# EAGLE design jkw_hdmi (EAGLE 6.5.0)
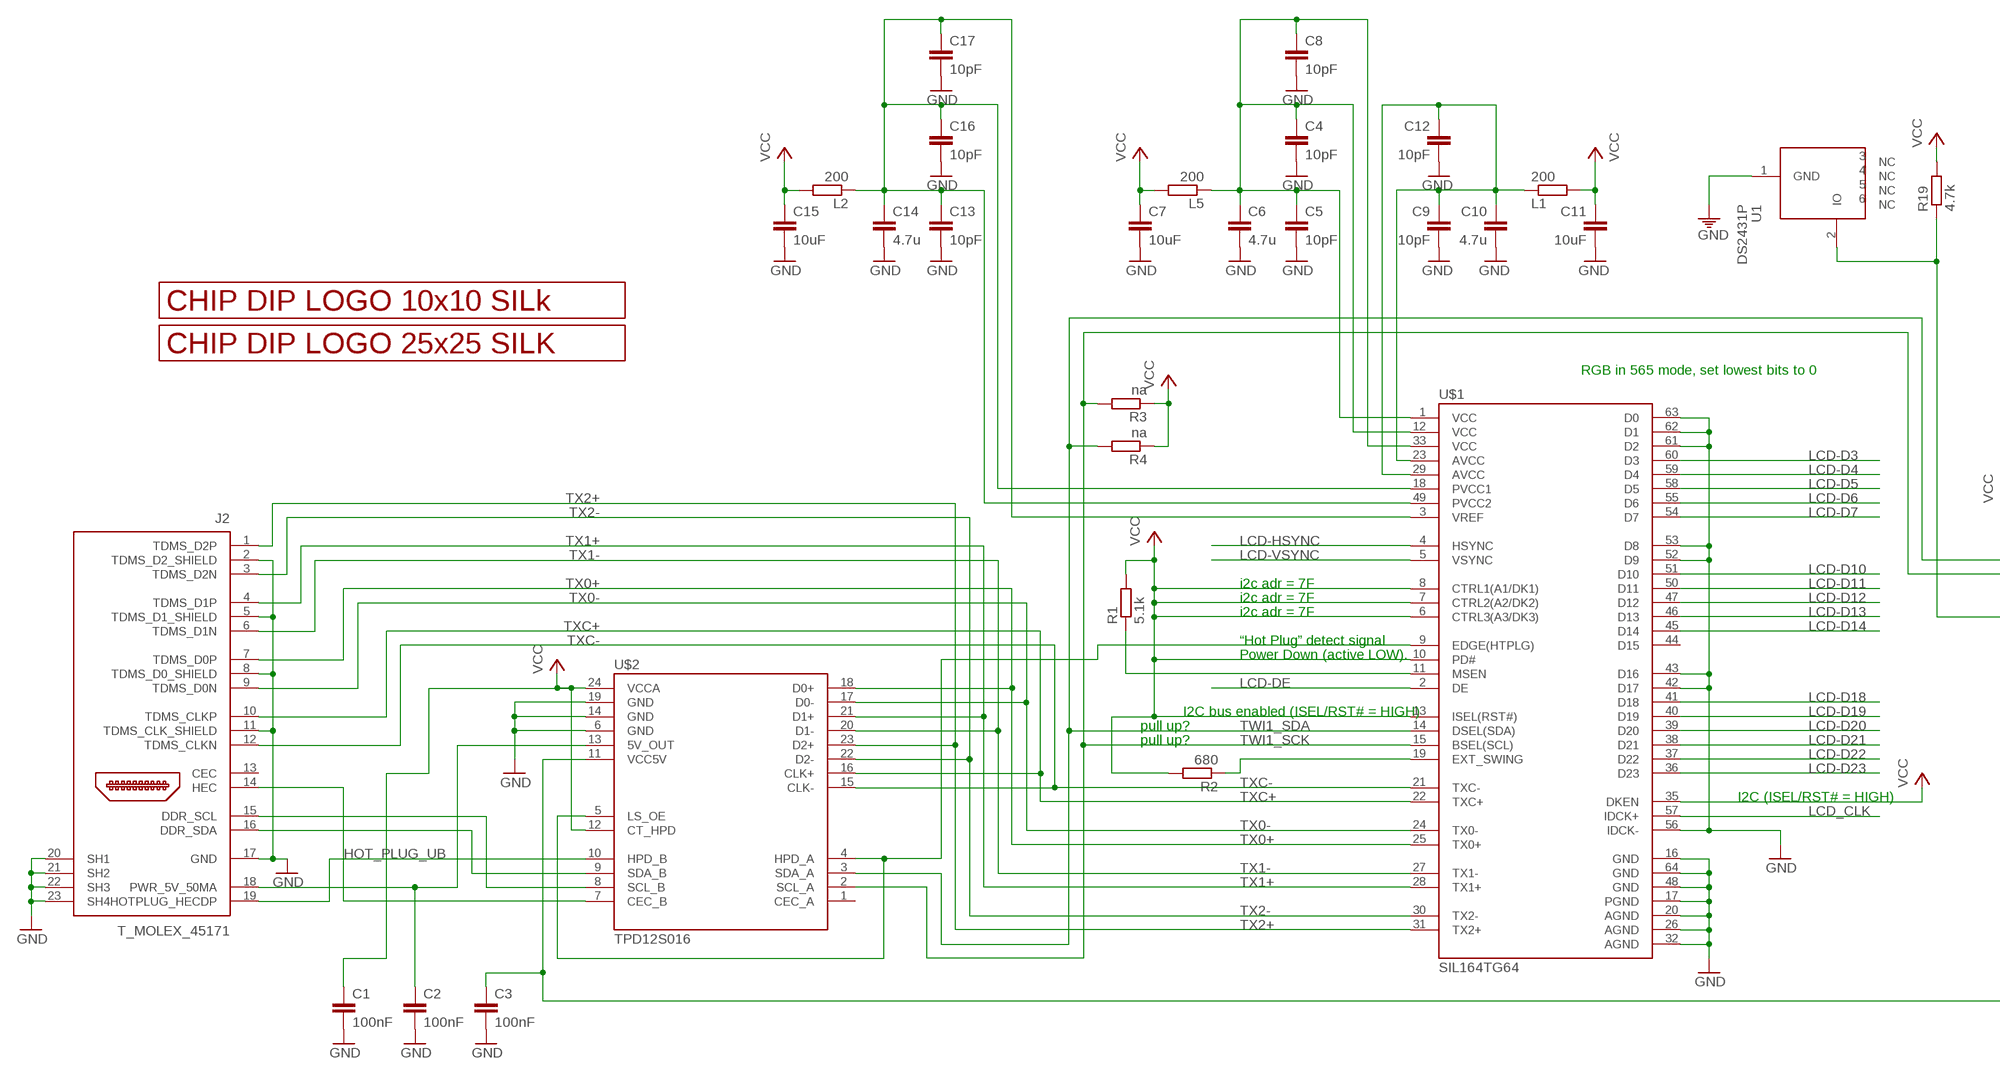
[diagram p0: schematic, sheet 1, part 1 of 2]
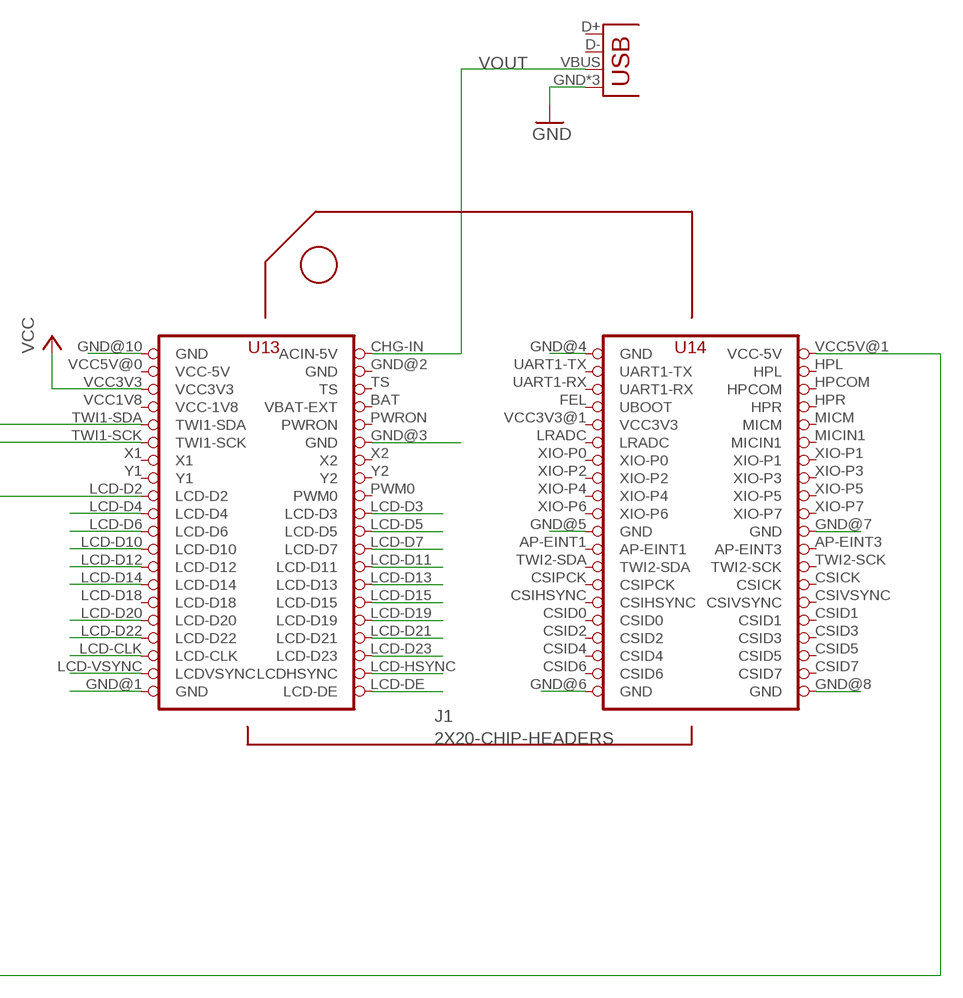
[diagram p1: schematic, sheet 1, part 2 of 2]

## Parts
C1  100nF  C-EUC0805  [C0805]
C2  100nF  C-EUC0805  [C0805]
C3  100nF  C-EUC0805  [C0805]
C4  10pF  C-EUC0805  [C0805]
C5  10pF  C-EUC0805  [C0805]
C6  4.7u  C-EUC0805  [C0805]
C7  10uF  C-EUC0805  [C0805]
C8  10pF  C-EUC0805  [C0805]
C9  10pF  C-EUC0805  [C0805]
C10  4.7u  C-EUC0805  [C0805]
C11  10uF  C-EUC0805  [C0805]
C12  10pF  C-EUC0805  [C0805]
C13  10pF  C-EUC0805  [C0805]
C14  4.7u  C-EUC0805  [C0805]
C15  10uF  C-EUC0805  [C0805]
C16  10pF  C-EUC0805  [C0805]
C17  10pF  C-EUC0805  [C0805]
J1  2X20-CHIP-HEADERS  [2X20CHIP_SM]
J2  T_MOLEX_45171  [T_MOLEX_45171]
L1  200  R-EU_R0805  [R0805]
L2  200  R-EU_R0805  [R0805]
L5  200  R-EU_R0805  [R0805]
POWER_USB  USBUSB-MICROB-SMT-DIP  [USB-MICROB-SMT-DIP]
R1  5.1k  R-EU_M0805  [M0805]
R2  680  R-EU_M0805  [M0805]
R3  na  R-EU_M0805  [M0805]
R4  na  R-EU_M0805  [M0805]
R19  4.7k  R-EU_R0805  [R0805]
U1  DS2431P  [TSOC6]
U$1  SIL164TG64  [TQFP64]
U$2  TPD12S016  [DIL24]
U$3  LOGO_10X10_SILK  [LOGO_10X10_SILK]
U$4  LOGO_25X25_SILK  [LOGO_25X25_SILK]

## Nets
ASD: R1.1 U$1.11(MSEN)
GND: C1.2 C2.2 C3.2 C4.2 C5.2 C6.2 C7.2 C8.2 C9.2 C10.2 C11.2 C12.2 C13.2 C14.2 C15.2 C16.2 C17.2 J1.GND@1(GND) J1.GND@3(GND) J1.GND@4(GND) J1.GND@5(GND) J1.GND@6(GND) J1.GND@7(GND) J1.GND@8(GND) J1.GND@10(GND) J2.2(TDMS_D2_SHIELD) J2.5(TDMS_D1_SHIELD) J2.8(TDMS_D0_SHIELD) J2.11(TDMS_CLK_SHIELD) J2.17(GND) J2.20(SH1) J2.21(SH2) J2.22(SH3) J2.23(SH4) POWER_USB.GND POWER_USB.MT1(GND) POWER_USB.MT2(GND) U1.1(GND) U$1.16(GND) U$1.17(PGND) U$1.20(AGND) U$1.26(AGND) U$1.32(AGND) U$1.42(D17) U$1.43(D16) U$1.48(GND) U$1.52(D9) U$1.53(D8) U$1.56(IDCK-) U$1.61(D2) U$1.62(D1) U$1.63(D0) U$1.64(GND) U$2.6(GND) U$2.14(GND) U$2.19(GND)
HOT_PLUG_UB: J2.19(HOTPLUG_HECDP) U$2.10(HPD_B)
HOTPLUG_DET: U$1.9(EDGE(HTPLG)) U$2.4(HPD_A) U$2.5(LS_OE)
LCD-D3: J1.LCD-D3 U$1.60(D3)
LCD-D4: J1.LCD-D4 U$1.59(D4)
LCD-D5: J1.LCD-D5 U$1.58(D5)
LCD-D6: J1.LCD-D6 U$1.55(D6)
LCD-D7: J1.LCD-D7 U$1.54(D7)
LCD-D10: J1.LCD-D10 U$1.51(D10)
LCD-D11: J1.LCD-D11 U$1.50(D11)
LCD-D12: J1.LCD-D12 U$1.47(D12)
LCD-D13: J1.LCD-D13 U$1.46(D13)
LCD-D14: J1.LCD-D14 U$1.45(D14)
LCD-D15: J1.LCD-D15
LCD-D18: U$1.41(D18)
LCD-D19: J1.LCD-D19 U$1.40(D19)
LCD-D20: J1.LCD-D20 U$1.39(D20)
LCD-D21: J1.LCD-D21 U$1.38(D21)
LCD-D22: J1.LCD-D22 U$1.37(D22)
LCD-D23: J1.LCD-D23 U$1.36(D23)
LCD-DE: J1.LCD-DE U$1.2(DE)
LCD-HSYNC: J1.LCD-HSYNC(LCDHSYNC) U$1.4(HSYNC)
LCD-VSYNC: J1.LCD-VSYNC(LCDVSYNC) U$1.5(VSYNC)
LCD_CLK: J1.LCD-CLK U$1.57(IDCK+)
N$2: R2.1 U$1.19(EXT_SWING)
N$3: C2.1 J2.18(PWR_5V_50MA) U$2.13(5V_OUT)
N$4: C4.1 C5.1 C6.1 C8.1 L5.1 U$1.1(VCC) U$1.12(VCC) U$1.33(VCC)
N$5: J1.LCD-D2 R19.1 U1.2(IO)
N$6: J2.15(DDR_SCL) U$2.8(SCL_B)
N$7: J2.16(DDR_SDA) U$2.9(SDA_B)
N$8: C9.1 C10.1 C12.1 L1.1 U$1.23(AVCC) U$1.29(AVCC)
N$9: J2.14(HEC) U$2.7(CEC_B)
N$10: C13.1 C14.1 C16.1 C17.1 L2.1 U$1.3(VREF) U$1.18(PVCC1) U$1.49(PVCC2)
TWI1_SCK: J1.TWI1-SCK R3.2 U$1.15(BSEL(SCL)) U$2.2(SCL_A)
TWI1_SDA: J1.TWI1-SDA R4.2 U$1.14(DSEL(SDA)) U$2.3(SDA_A)
TX0+: J2.7(TDMS_D0P) U$1.25(TX0+) U$2.18(D0+)
TX0-: J2.9(TDMS_D0N) U$1.24(TX0-) U$2.17(D0-)
TX1+: J2.4(TDMS_D1P) U$1.28(TX1+) U$2.21(D1+)
TX1-: J2.6(TDMS_D1N) U$1.27(TX1-) U$2.20(D1-)
TX2+: J2.1(TDMS_D2P) U$1.31(TX2+) U$2.23(D2+)
TX2-: J2.3(TDMS_D2N) U$1.30(TX2-) U$2.22(D2-)
TXC+: J2.10(TDMS_CLKP) U$1.22(TXC+) U$2.16(CLK+)
TXC-: J2.12(TDMS_CLKN) U$1.21(TXC-) U$2.15(CLK-)
VCC: C1.1 C7.1 C11.1 C15.1 J1.VCC3V3 L1.2 L2.2 L5.2 R1.2 R2.2 R3.1 R4.1 R19.2 U$1.6(CTRL3(A3/DK3)) U$1.7(CTRL2(A2/DK2)) U$1.8(CTRL1(A1/DK1)) U$1.10(PD#) U$1.13(ISEL(RST#)) U$1.35(DKEN) U$2.12(CT_HPD) U$2.24(VCCA)
VCC_5V_DCC: C3.1 J1.VCC5V@1(VCC-5V) U$2.11(VCC5V)
VOUT: J1.CHG-IN(ACIN-5V) POWER_USB.VBUS
Unconnected: J1.AP-EINT1 J1.AP-EINT3 J1.BAT(VBAT-EXT) J1.CSICK J1.CSID0 J1.CSID1 J1.CSID2 J1.CSID3 J1.CSID4 J1.CSID5 J1.CSID6 J1.CSID7 J1.CSIHSYNC J1.CSIPCK J1.CSIVSYNC J1.FEL(UBOOT) J1.HPCOM J1.HPL J1.HPR J1.LCD-D18 J1.LRADC J1.MICIN1 J1.MICM J1.PWM0 J1.PWRON J1.TS J1.TWI2-SCK J1.TWI2-SDA J1.UART1-RX J1.UART1-TX J1.X1 J1.X2 J1.XIO-P0 J1.XIO-P1 J1.XIO-P2 J1.XIO-P3 J1.XIO-P4 J1.XIO-P5 J1.XIO-P6 J1.XIO-P7 J1.Y1 J1.Y2 J2.13(CEC) POWER_USB.D+ POWER_USB.D- U1.3(NC) U1.4(NC) U1.5(NC) U1.6(NC) U$2.1(CEC_A)

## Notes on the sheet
- RGB in 565 mode, set lowest bits to 0
- i2c adr = 7F
- i2c adr = 7F
- i2c adr = 7F
- “Hot Plug” detect signal
- Power Down (active LOW).
- I2C bus enabled (ISEL/RST# = HIGH)
- pull up?
- pull up?
- I2C (ISEL/RST# = HIGH)

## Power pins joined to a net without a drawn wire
D15: U$1.44(D15)
GND: J1.GND@2(GND)
VCC3V3: J1.VCC3V3@1(VCC3V3)
VCC-1V8: J1.VCC1V8(VCC-1V8)
VCC-5V: J1.VCC5V@0(VCC-5V)

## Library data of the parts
C1-C17 = rcl:C-EU: CAPACITOR, European symbol
J1 = VGA-DIP:2X20-CHIP-HEADERS: Through hole layout with chip reference
J2 = CHIP_HDMI:T_MOLEX_45171
L1 L2 L5 R1-R4 R19 = rcl:R-EU_: RESISTOR, European symbol
POWER_USB = Spark:USB
U1 = VGA-DIP:DS2431: 1024-Bit EEPROM This chip provides a 4x256 Bit EEPROM, which can be programmed@5V. Write protection and OTP emulation are available, too. Author: Jan Kandziora <jjj@gmx.de>; DESCRIPTION: IC, 1024-Bit, 1-Wire EEPROM, TSOC6; FOOTPRINT: TSOC6; LINK: http://www.digikey.com/product-detail/en/DS2431P%2BT%26R/DS2431P%2BT%26RCT-ND/3647900; MFG: DIGIKEY; MFG_PN: DS2431P+T&RCT-ND; PART_TYPE: IC; PRICE: 0.98; VENDOR: MAXIM; VENDOR_PART_NUMBER: DS2431P+T&R
U$1 = SII164CTG64:SIL164TG64
U$2 = SII164CTG64:TPD12S016
U$3 = logo:LOGO_10X10_SILK
U$4 = logo:LOGO_25X25_SILK

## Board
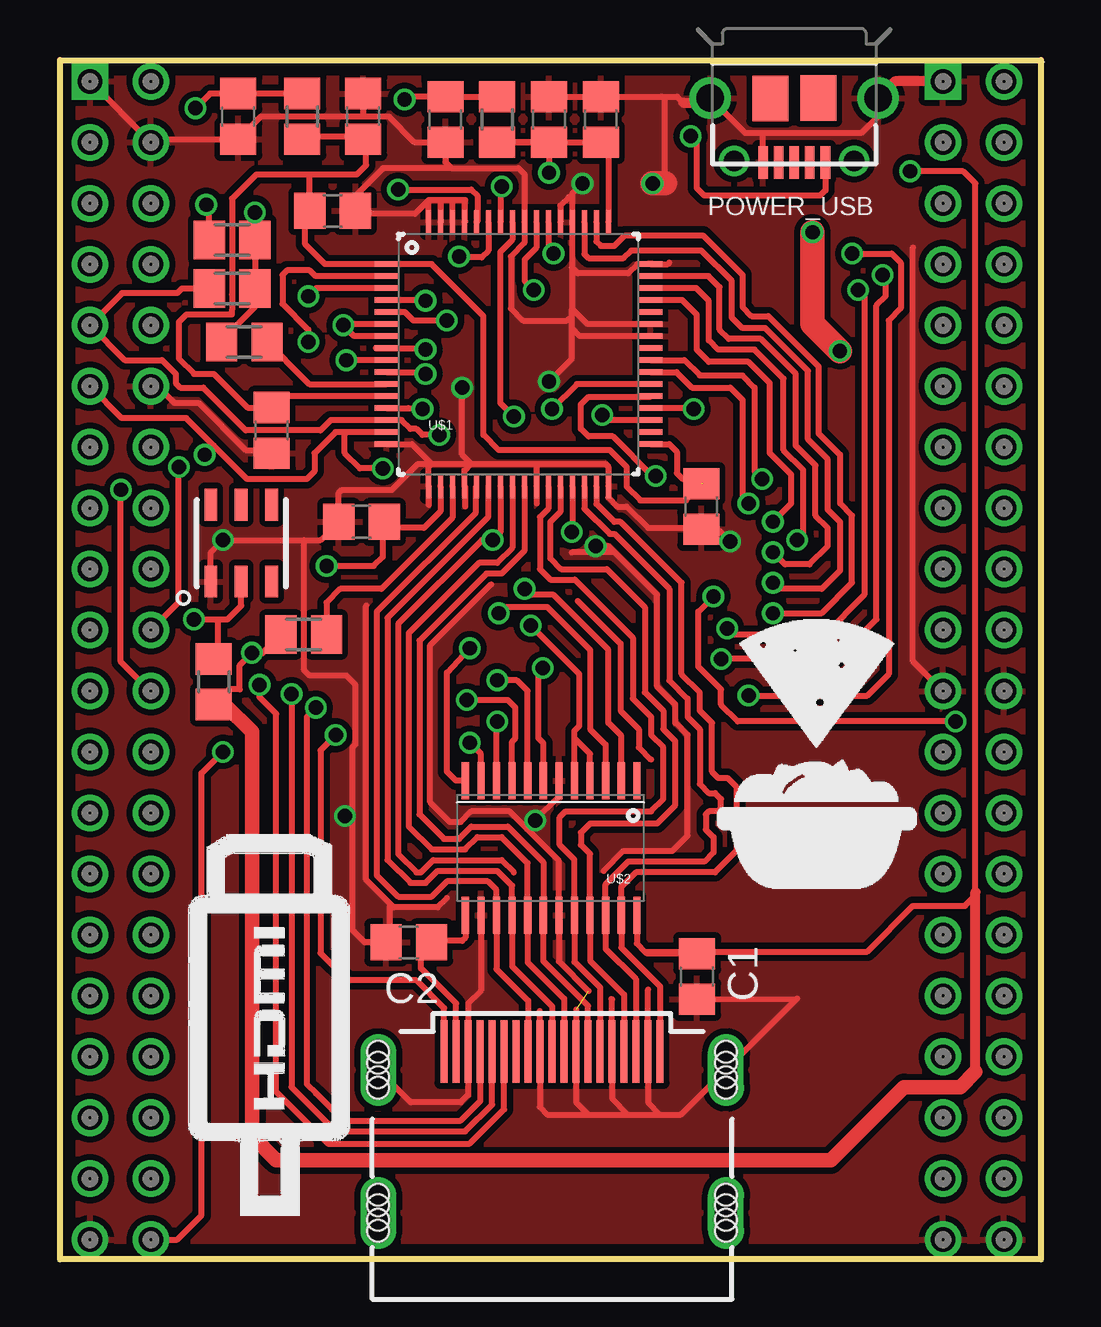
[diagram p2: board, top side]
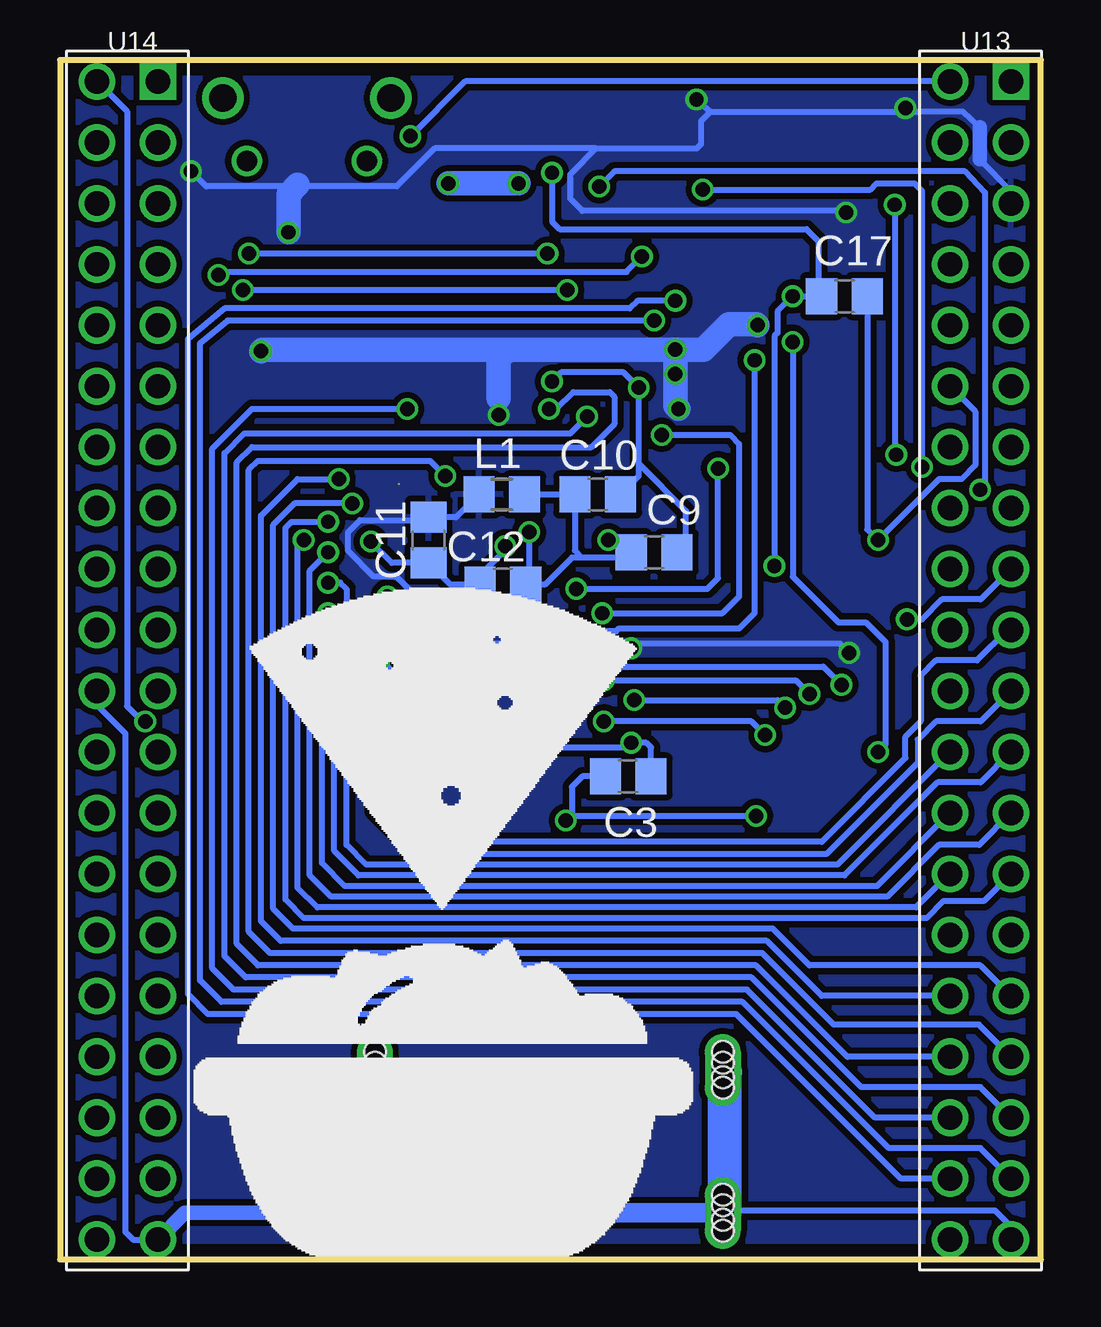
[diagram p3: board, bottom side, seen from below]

Size 40.89 x 49.97 mm. Coordinates in mm from the lower left corner, seen from the top.
Outline: 0,49.97 40.89,49.97 40.89,0 0,0 0,49.97
Copper layers (1*16): Top 0.035mm / dielectric 1.6mm / Bottom 0.035mm
Design rules "Elecrow_2-layer_PCB_eagle_rule": minimum track width 6mil, minimum drill 12mil, track to track 6mil, track to pad 6mil, pad to pad 6mil, via to via 8mil, smd to smd 0mil, copper to edge 20mil, drill to drill 10mil, minimum pad ring 6mil, minimum via ring 6mil, stop-mask expansion 0mil, vias tented up to drill 100mil, thermal gap 10mil

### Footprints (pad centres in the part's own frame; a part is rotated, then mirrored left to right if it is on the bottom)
C0805 = smd 1.3 x 1.5: 1 -0.95,0; 2 0.95,0
2X20CHIP_SM = drill 1.016: AP-EINT1 36.81,21.65; AP-EINT3 39.35,21.65; BAT 3.79,41.97; CHG-IN 3.79,49.59; CSICK 39.35,16.57; CSID0 36.81,11.49; CSID1 39.35,11.49; CSID2 36.81,8.95; CSID3 39.35,8.95; CSID4 36.81,6.41; CSID5 39.35,6.41; CSID6 36.81,3.87; CSID7 39.35,3.87; CSIHSYNC 36.81,14.03; CSIPCK 36.81,16.57; CSIVSYNC 39.35,14.03; FEL 36.81,41.97; GND@1 3.79,36.89; GND@2 1.25,1.33; GND@4 39.35,24.19; GND@5 39.35,1.33; GND@6 36.81,1.33; GND@7 36.81,24.19; GND@10 3.79,47.05; HPCOM 39.35,44.51; HPL 39.35,47.05; HPR 39.35,41.97; LCD-CLK 1.25,6.41; LCD-D2 1.25,29.27; LCD-D3 3.79,26.73; LCD-D4 1.25,26.73; LCD-D5 3.79,24.19; LCD-D6 1.25,24.19; LCD-D7 3.79,21.65; LCD-D10 1.25,21.65; LCD-D11 3.79,19.11; LCD-D12 1.25,19.11; LCD-D13 3.79,16.57; LCD-D14 1.25,16.57; LCD-D15 3.79,14.03; LCD-D18 1.25,14.03; LCD-D19 3.79,11.49; LCD-D20 1.25,11.49; LCD-D21 3.79,8.95; LCD-D22 1.25,8.95; LCD-D23 3.79,6.41; LCD-DE 3.79,1.33; LCD-HSYNC 3.79,3.87; LCD-VSYNC 1.25,3.87; LRADC 36.81,36.89; MICIN1 39.35,36.89; MICM 39.35,39.43; PWM0 3.79,29.27; PWRON 3.79,39.43; TS 3.79,44.51; TWI1-SCK 1.25,36.89; TWI1-SDA 1.25,39.43; TWI2-SCK 39.35,19.11; TWI2-SDA 36.81,19.11; UART1-RX 36.81,44.51; UART1-TX 36.81,47.05; VCC1V8 1.25,41.97; VCC3V3 1.25,44.51; VCC3V3@1 36.81,39.43; VCC5V@0 1.25,47.05; VCC5V@1 39.35,49.59; X1 1.25,34.35; X2 3.79,34.35; XIO-P0 36.81,34.35; XIO-P1 39.35,34.35; XIO-P2 36.81,31.81; XIO-P3 39.35,31.81; XIO-P4 36.81,29.27; XIO-P5 39.35,29.27; XIO-P6 36.81,26.73; XIO-P7 39.35,26.73; Y1 1.25,31.81; Y2 3.79,31.81 | drill 1.016 square: GND@3 1.25,49.59; GND@8 36.81,49.59
T_MOLEX_45171 = smd 0.3 x 2.6: 1 4.5,10.31; 2 4,10.31; 3 3.5,10.31; 4 3,10.31; 5 2.5,10.31; 6 2,10.31; 7 1.5,10.31; 8 1,10.31; 9 0.5,10.31; 10 0,10.31; 11 -0.5,10.31; 12 -1,10.31; 13 -1.5,10.31; 14 -2,10.31; 15 -2.5,10.31; 16 -3,10.31; 17 -3.5,10.31; 18 -4,10.31; 19 -4.5,10.31 | drill 0.9 pad 1.499 long: 20 -7.25,3.59; 21 7.25,3.59; 22 7.25,9.55; 23 -7.25,9.55 | hole 0.9: -7.25,10.3; -7.25,8.8; -7.25,9.85; -7.25,9.25; -7.25,4.35; -7.25,2.85; -7.25,3.9; -7.25,3.3; 7.25,10.3; 7.25,8.8; 7.25,9.85; 7.25,9.25; 7.25,4.35; 7.25,3.9; 7.25,2.85; 7.25,3.3
R0805 = smd 1.3 x 1.5: 1 -0.95,0; 2 0.95,0
USB-MICROB-SMT-DIP = smd 0.4 x 1.35: D+ 0,2.675; D- -0.65,2.675; GND 1.3,2.675; ID 0.65,2.675; VBUS -1.3,2.675 | drill 1.15 pad 1.7: MT1 -3.5,0; MT2 3.5,0 | drill 0.85 pad 1.25: MT3 -2.5,2.625; MT4 2.5,2.625 | smd 1.5 x 1.9: P$1 -1,0; P$2 1,0.01
M0805 = smd 1.3 x 1.6: 1 -0.95,0; 2 0.95,0
TSOC6 = smd 0.53 x 1.33: 1 -1.27,-1.6; 2 0,-1.6; 3 1.27,-1.6; 4 1.27,1.6; 5 0,1.6; 6 -1.27,1.6
TQFP64 = smd 1 x 0.22: 1 -5.5,3.75; 2 -5.5,3.25; 3 -5.5,2.75; 4 -5.5,2.25; 5 -5.5,1.75; 6 -5.5,1.25; 7 -5.5,0.75; 8 -5.5,0.25; 9 -5.5,-0.25; 10 -5.5,-0.75; 11 -5.5,-1.25; 12 -5.5,-1.75; 13 -5.5,-2.25; 14 -5.5,-2.75; 15 -5.5,-3.25; 16 -5.5,-3.75; 33 5.5,-3.75; 34 5.5,-3.25; 35 5.5,-2.75; 36 5.5,-2.25; 37 5.5,-1.75; 38 5.5,-1.25; 39 5.5,-0.75; 40 5.5,-0.25; 41 5.5,0.25; 42 5.5,0.75; 43 5.5,1.25; 44 5.5,1.75; 45 5.5,2.25; 46 5.5,2.75; 47 5.5,3.25; 48 5.5,3.75 | smd 0.22 x 1: 17 -3.75,-5.5; 18 -3.25,-5.5; 19 -2.75,-5.5; 20 -2.25,-5.5; 21 -1.75,-5.5; 22 -1.25,-5.5; 23 -0.75,-5.5; 24 -0.25,-5.5; 25 0.25,-5.5; 26 0.75,-5.5; 27 1.25,-5.5; 28 1.75,-5.5; 29 2.25,-5.5; 30 2.75,-5.5; 31 3.25,-5.5; 32 3.75,-5.5; 49 3.75,5.5; 50 3.25,5.5; 51 2.75,5.5; 52 2.25,5.5; 53 1.75,5.5; 54 1.25,5.5; 55 0.75,5.5; 56 0.25,5.5; 57 -0.25,5.5; 58 -0.75,5.5; 59 -1.25,5.5; 60 -1.75,5.5; 61 -2.25,5.5; 62 -2.75,5.5; 63 -3.25,5.5; 64 -3.75,5.5
DIL24 = smd 0.3 x 1.55: 1 -3.6,-2.8; 2 -2.95,-2.8; 3 -2.3,-2.8; 4 -1.65,-2.8; 5 -1,-2.8; 6 -0.35,-2.8; 7 0.3,-2.8; 8 0.95,-2.8; 9 1.6,-2.8; 10 2.25,-2.8; 11 2.9,-2.8; 12 3.55,-2.8; 13 3.55,2.8; 14 2.9,2.8; 15 2.25,2.8; 16 1.6,2.8; 17 0.95,2.8; 18 0.3,2.8; 19 -0.35,2.8; 20 -1,2.8; 21 -1.65,2.8; 22 -2.3,2.8; 23 -2.95,2.8; 24 -3.6,2.8

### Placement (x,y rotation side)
C1  26.56,11.79 270 top
C2  14.54,13.21 180 top
C3  17.21,20.13 180 bottom
C4  8.83,34.54 270 top
C5  11.37,43.69 0 top
C6  12.64,47.62 90 top
C7  7.43,47.62 270 top
C8  26.73,31.37 270 top
C9  16.13,29.46 0 bottom
C10  18.48,31.88 0 bottom
C11  25.53,29.97 270 bottom
C12  22.43,28.12 180 bottom
C13  22.54,47.5 90 top
C14  20.38,47.5 90 top
C15  16.07,47.5 270 top
C16  12.57,30.73 180 top
C17  8.19,40.13 0 bottom
J1  0,-0.51 0 top
J2  20.51,-1.65 0 top
L1  22.48,31.88 180 bottom
L2  18.22,47.5 90 top
L5  10.1,47.62 90 top
POWER_USB  30.61,48.39 180 top
R1  7.68,38.23 180 top
R2  10.16,26.04 180 top
R3  7.18,42.48 180 top
R4  7.18,40.45 180 top
R19  6.41,24.07 270 top
U1  7.56,29.84 0 top
U$1  19.11,37.72 0 top
U$2  20.45,17.15 180 top
U$3  27.37,15.43 0 top
U$4  35.37,-0.13 0 bottom

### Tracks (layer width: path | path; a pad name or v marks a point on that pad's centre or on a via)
ASD
  Top 0.254: R1.1 8.45,38.42 10.39,36.47 U$1.11
GND  (via drill 0.6)  (1 unrouted)
  Top 0.254: C14.2 C13.2 25.08,48.45 | 24.51,11.24 J2.2 24.51,6.54 25.02,6.03 | J2.11 | J2.11 20,10.35 | 21.53,10.41 21.53,8.68 J2.8 21.51,6.56 22.04,6.03 | 22.99,10.86 23.01,10.84 J2.5 23.01,6.71 23.69,6.03 | 22.04,11.18 20.8,12.41 U$2.19 20.8,16.6 19.46,17.94 | 19.88,31.5 19.88,32.21 | 19.88,32.21 U$1.26 | 17.97,28.13 15.43,25.59 15.43,19.05 16.26,18.23 16.7,18.23 17.14,18.67 18.73,18.67 19.46,17.94 | 20.83,19.91 U$2.6 20.8,19.27 v19.81,18.29 19.46,17.94 | J2.23 14.62,6.54 16.7,6.54 17.01,6.85 J2.17 17.02,10.67 17.55,11.2 U$2.14 | 25.4,41.53 25.34,41.47 U$1.48 24.07,41.47 23.69,41.09 21.59,41.09 21.34,41.34 21.36,41.37 | U$1.52 21.36,44.11 21.21,44.26 20.86,43.91 U$1.53 | U$1.61 16.89,43.25 16.89,44.13 16.32,44.13 | U$1.63 15.88,43.23 15.88,44.13 | 16.32,44.13 15.88,44.13 | 15.88,44.13 15.37,44.13 15.36,44.13 | 16.89,31.37 16.89,32.19 U$1.20 16.86,32.87 17.14,33.15 | 15.37,31.43 U$1.17 15.36,33.02 15.49,33.15 | J1.GND@1 4.07,36.38 4.76,35.69 5.78,35.69 7.75,33.72 8.7,33.72 C4.2 | 27.94,8.08 J2.22 | 19.88,32.21 19.88,33.08 19.94,33.15 | 19.94,33.15 22.73,33.15 22.86,33.02 U$1.32 22.86,31.75 23.24,31.37 23.62,31.37 24.51,30.48 26.67,30.48 C8.2 26.8,30.35 27.49,30.35 v27.94,29.91 | 17.14,33.15 19.94,33.15 | U$1.16 14.67,33.97 15.49,33.15 | U$1.64 15.36,44.13 | U$1.52 21.36,44.41 v21.78,44.83 | 21.36,41.37 U$1.52 | U$1.43 21.99,38.97 21.36,39.6 | 21.36,39.6 21.36,41.37 | U$1.42 21.67,38.47 21.34,38.8 | 21.34,38.8 21.34,39.31 | 21.34,39.31 21.34,39.57 21.36,39.6 | 17.14,33.15 16.76,33.53 v16.76,36.32 | v20.38,36.58 21.34,37.53 21.34,38.8 | 15.49,33.15 17.14,33.15 | 25.08,48.45 25.72,48.45 25.97,48.2 | 15.36,44.13 14.8,43.56 12.44,43.56 C5.2 12.32,44.32 13.46,45.47 16.32,45.47
  Top 0.254: 16.32,45.47 16.07,45.72 C15.2 14.77,46.55 13.69,47.62 12.7,47.62 | 16.32,45.47 19.11,45.47 19.37,45.21 U$1.56 19.36,42.35 18.8,41.78 18.8,39.62 19.3,39.12 21.15,39.12 21.34,39.31 | 12.7,47.62 8.38,47.62 C7.2 3.92,46.68 J1.GND@10 J1.GND@3 | C6.2 12.64,47.69 12.7,47.62 | U$1.62 16.36,44.09 16.32,44.13 | U1.1 6.29,29.46 v6.79,29.97 10.16,29.97 | 10.16,29.97 10.86,29.97 C16.2 11.62,31.94 11.75,32.07 13.84,32.07 14.92,33.15 15.49,33.15 | J2.11 20,6.35 20.32,6.03 22.04,6.03 | 22.04,6.03 23.69,6.03 | 23.69,6.03 25.02,6.03 | 25.02,6.03 25.89,6.03 J2.22 | 10.16,29.97 10.16,24.57 10.41,24.32 11.94,24.32 12.32,23.94 12.32,21.46 12.19,21.34 12.19,13.72 12.7,13.21 C2.2 13.75,13.37 13.75,14.82 | C1.2 30.72,10.86 J2.22 | J1.GND@7 35.56,24.93 35.56,42.16 | POWER_USB.MT1 34.11,47.63 33.4,46.93 29.34,46.93 | 29.34,46.93 28.57,46.93 POWER_USB.MT2 | POWER_USB.GND 29.31,46.9 29.34,46.93 | 25.21,44.83 25.21,48.32 25.08,48.45 | 16.13,15.05 15.75,14.67 13.91,14.67 13.75,14.82 | 13.75,14.82 12.76,15.81 12.76,27.24 | 22.67,16.19 23.49,17.02 25.53,17.02 26.16,17.65 26.16,21.84 25.65,22.35 25.65,23.11 24.89,23.88 24.89,27.69 23.11,29.46 | 23.11,29.46 21.34,29.46 | 23.11,29.46 22.86,29.72 v22.33,29.72
  Top 0.406: 25.97,48.2 27.11,48.2 POWER_USB.MT2 | J1.GND@8 34.8,49.08 POWER_USB.MT1
  Top 1.016: v24.7,44.83 25.21,44.83
  Bottom 0.254: J1.GND@2 1.25,1.38 1.91,2.03 13.17,2.03 J2.20 | J1.GND@6 37.85,0.82 38.16,1.14 38.16,21.91 39.35,23.09 J1.GND@4 | 13.17,7.81 J2.23 | C3.2 19.11,20.13 19.56,19.69 19.56,18.54 19.62,18.48 | v20.38,36.58 20,36.96 17.4,36.96 v16.76,36.32 16.76,33.15 | C10.2 16.76,32.64 16.76,33.15 | C9.2 14.8,29.85 14.8,31.18 16.76,33.15 | C17.2 7.24,30.42 v6.79,29.97 4.25,32.51 3.3,32.51 2.74,33.08 2.74,35.34 J1.GND@1 | 25.21,28.7 C11.2 | C11.2 27.05,29.02 v27.94,29.91 | 19.62,18.48 v19.81,18.29 | 19.62,18.48 v11.88,18.48 | 23.38,28.6 23.38,28.51 | C11.2 24.62,28.12 C12.2 23.38,28.51 | 23.38,28.51 22.33,29.56 v22.33,29.72
  Bottom 0.61: J2.21 35.69,1.94 J1.GND@6
  Bottom 0.813: J2.20 J2.21
  Bottom 1.016: v21.78,44.83 v24.7,44.83
  Bottom 1.422: J2.21 J2.22 | 13.17,2.03 13.17,7.81
  pour Top (isolate 0.254): 0.13,0 40.89,0 40.89,50 0.13,50
HOT_PLUG_UB  (via drill 0.6)
  Top 0.254: J2.19 16.01,10.47 14.86,11.62 12,11.62 10.86,12.76 10.86,21.21 v11.49,21.84 | U$2.10 18.2,22.39 v18.22,22.41
  Bottom 0.254: v11.49,21.84 12.07,22.41 v18.22,22.41
HOTPLUG_DET  (via drill 0.6)
  Top 0.254: U$2.5 21.45,21.72 | U$2.4 22.1,21.07 21.45,21.72 | U$1.9 v11.94,37.47 | v19.62,26.42 21.65,24.38 21.65,22.23 21.45,22.02 21.45,21.72
  Bottom 0.254: v11.94,37.47 11.94,26.92 12.57,26.29 17.59,26.29 17.72,26.16 19.37,26.16 v19.62,26.42
LCD-D3  (via drill 0.6)
  Top 0.254: J1.LCD-D3 4.95,27.38 v4.95,33.02 | v14.1,44.58 17.14,44.58 17.4,44.32 17.4,43.25 U$1.60
  Bottom 0.254: v4.95,33.02 4.95,44.51 5.27,44.83 6.86,44.83 7.11,44.58 v14.1,44.58
LCD-D4  (via drill 0.6)
  Top 0.254: v34.29,41.02 34.42,40.89 34.42,40.13 34.04,39.75 34.04,26.67 32.38,25.02 v27.56,25.02 | U$1.59 17.86,42.03 17.58,41.75 16.67,41.75 v16.64,41.78
  Bottom 0.254: J1.LCD-D4 1.4,26.22 2.67,24.95 4.38,24.95 5.02,24.32 5.02,22.41 5.65,21.78 5.65,20.89 9.14,17.4 24.38,17.4 26.8,19.81 26.8,24.26 v27.56,25.02 | v34.29,41.02 34.16,41.15 17.27,41.15 v16.64,41.78
LCD-D5  (via drill 0.6)
  Top 0.254: v2.54,32.07 2.54,24.89 3.75,23.68 J1.LCD-D5 | v18.41,44.7 18.36,44.65 U$1.58
  Bottom 0.254: v18.41,44.7 17.78,45.34 3.18,45.34 2.34,44.45 2.34,32.27 v2.54,32.07
LCD-D6  (via drill 0.6)
  Top 0.254: v33.27,40.39 33.4,40.39 33.53,40.26 33.53,27.69 31.88,26.04 28.07,26.04 v27.81,26.29 | U$1.55 19.86,42.15 19.37,41.66 19.37,40.77 v19.75,40.39 19.43,40.7
  Bottom 0.254: J1.LCD-D6 2.52,22.41 4.38,22.41 5.14,21.65 5.14,20.7 8.95,16.89 26.04,16.89 27.81,18.67 27.81,24 28.58,24.77 28.58,25.4 27.81,26.16 v27.81,26.29 | v19.75,40.39 v33.27,40.39
LCD-D7  (via drill 0.6)
  Top 0.254: v28.7,23.49 33.66,23.49 34.54,24.38 34.54,39.12 35.05,39.62 35.05,41.53 34.67,41.91 v33.02,41.91 | U$1.54 20.36,42.12 v20.57,41.91
  Bottom 0.254: J1.LCD-D7 8.49,16.45 28.13,16.45 28.96,17.27 28.96,23.24 v28.7,23.49 | v20.57,41.91 v33.02,41.91
LCD-D10  (via drill 0.6)
  Top 0.254: U$1.51 21.86,41.89 22.04,41.72 23.49,41.72 23.81,42.04 26.73,42.04 28,40.77 28,39.24 28.45,38.8 29.4,38.8 31.18,37.02 31.18,34.16 32,33.34 32,31.24 32.51,30.73 32.51,28.7 31.75,27.94 29.97,27.94 v29.72,28.19
  Bottom 0.254: J1.LCD-D10 2.52,19.88 4.32,19.88 8.19,16 28.45,16 29.46,17.02 29.46,25.91 28.96,26.42 28.96,27.94 29.21,28.19 v29.72,28.19
LCD-D11  (via drill 0.6)
  Top 0.254: U$1.50 22.36,42.41 22.54,42.23 23.11,42.23 23.56,42.67 26.8,42.67 28.45,41.02 28.45,39.69 28.83,39.31 29.53,39.31 31.62,37.21 31.62,34.42 32.51,33.53 32.51,31.5 33.02,30.99 33.02,28.19 31.75,26.92 v29.72,26.92
  Bottom 0.254: J1.LCD-D11 6.84,15.56 29.02,15.56 29.97,16.51 29.97,26.67 v29.72,26.92
LCD-D12  (via drill 0.6)
  Top 0.254: v29.72,29.46 30.23,28.96 31.24,28.96 32,29.72 32,30.48 31.5,30.99 31.5,33.08 30.67,33.91 30.67,36.89 29.21,38.35 27.88,38.35 27.49,38.73 27.49,40.51 27.04,40.97 U$1.47
  Bottom 0.254: J1.LCD-D12 2.58,17.27 4.25,17.27 6.41,15.11 29.59,15.11 30.48,16 30.48,28.7 v29.72,29.46
LCD-D13  (via drill 0.6)
  Top 0.254: v30.73,29.97 30.99,30.23 30.99,32.89 30.16,33.72 30.16,36.7 28.96,37.91 27.43,37.91 27.05,38.29 27.05,39.94 26.52,40.47 U$1.46
  Bottom 0.254: J1.LCD-D13 3.81,16.06 5.21,14.67 30.16,14.67 30.99,15.49 30.99,29.72 v30.73,29.97
LCD-D14  (via drill 0.6)
  Top 0.254: v29.72,30.73 30.48,31.5 30.48,32.7 29.59,33.59 29.59,36.51 28.7,37.4 27.05,37.4 26.54,37.91 26.54,39.37 25.94,39.97 U$1.45
  Bottom 0.254: J1.LCD-D14 2.39,14.92 4.06,14.92 4.76,14.22 30.73,14.22 31.5,14.99 31.5,30.48 31.24,30.73 v29.72,30.73
LCD-D19  (via drill 0.6)
  Top 0.254: U$1.40 26.03,37.47 26.67,36.83 28.45,36.83 28.96,36.32 28.96,32.83 v29.27,32.51
  Bottom 0.254: J1.LCD-D19 9.14,10.98 11.43,13.27 31.69,13.27 32.51,14.1 32.51,30.99 30.99,32.51 v29.27,32.51
LCD-D20  (via drill 0.6)
  Top 0.254: U$1.39 25.71,36.97 26.35,36.32 27.94,36.32 28.45,35.81 28.45,31.75 v28.7,31.5
  Bottom 0.254: J1.LCD-D20 2.52,12.26 9.65,12.26 11.18,13.78 31.18,13.78 32,14.6 32,30.61 31.12,31.5 v28.7,31.5
LCD-D21  (via drill 0.6)
  Top 0.254: U$1.38 21.55,36.47 v20.51,35.43
  Bottom 0.254: J1.LCD-D21 8.06,8.44 11.88,12.26 32.64,12.26 33.53,13.14 33.53,33.21 32.89,33.84 18.73,33.84 17.78,34.8 17.78,35.94 17.97,36.13 19.49,36.13 20.19,35.43 v20.51,35.43
LCD-D22  (via drill 0.6)
  Top 0.254: 24.77,32.7 v24.83,32.64 24.7,32.64 23.05,34.29 22.04,34.29 21.72,34.61 21.72,35.62 22.04,35.94 24.59,35.94 U$1.37
  Bottom 0.254: J1.LCD-D22 2.59,9.78 8.64,9.78 11.62,12.76 32.13,12.76 33.02,13.65 33.02,32.89 32.64,33.27 25.46,33.27 v24.83,32.64
LCD-D23  (via drill 0.6)
  Top 0.254: v26.42,35.43 26.38,35.47 U$1.36
  Bottom 0.254: J1.LCD-D23 6.92,5.9 12.26,11.24 33.66,11.24 34.54,12.13 34.54,33.78 32.89,35.43 v26.42,35.43
LCD-DE  (via drill 0.6)
  Top 0.254: U$1.2 10.66,40.97 10.41,41.21 9.46,41.21 9.27,41.02 9.27,39.82 10.35,38.73 v10.35,38.23 | J1.LCD-DE 4.89,0.82 5.91,1.84 5.91,20.26 v6.79,21.15
  Bottom 0.254: v10.35,38.23 10.35,28.45 8.45,26.54 7.3,26.54 6.48,25.72 6.48,21.46 v6.79,21.15
LCD-HSYNC  (via drill 0.6)
  Top 0.254: v15.24,39.94 15.21,39.97 U$1.4
  Bottom 0.254: J1.LCD-HSYNC 5.84,3.36 12.7,10.22 34.73,10.22 35.56,11.05 35.56,38.35 34.04,39.62 17.14,39.62 16.83,39.94 v15.24,39.94
LCD-VSYNC  (via drill 0.6)
  Top 0.254: v16.13,39.12 14.73,39.12 14.38,39.47 U$1.5
  Bottom 0.254: J1.LCD-VSYNC 2.52,4.64 6.35,4.64 12.45,10.73 34.16,10.73 35.05,11.62 35.05,38.16 33.91,39.12 v16.13,39.12
LCD_CLK  (via drill 0.6)
  Top 0.254: 18.86,35.18 v18.92,35.12 18.35,35.69 18.35,41.97 18.86,42.48 U$1.57
  Bottom 0.254: J1.LCD-CLK 2.52,7.18 7.49,7.18 12.07,11.75 33.15,11.75 34.04,12.64 34.04,33.59 33.21,34.42 19.62,34.42 v18.92,35.12
N$2
  Top 0.254: U$1.19 16.36,30.91 13.4,27.94 11.68,27.94 11.11,27.37 R2.1
N$3
  Top 0.254: U$2.13 16.9,13.4 16.76,13.27 15.5,13.27 C2.1 15.05,13.21 15.05,12.13 16.51,10.67 J2.18
N$4  (1 unrouted)
  Top 0.254: U$1.33 25.4,33.97 25.72,33.66 25.72,32.77 25.97,32.51 26.54,32.51 C8.1 | U$1.12 9.3,35.97 C4.1 7.81,35.49 6.41,36.89 5.59,36.89 4.95,37.53 4.95,39.05 5.27,39.37 7.18,39.37 7.18,39.56 7.18,40.2 7.18,44.2 8.19,45.21 10.41,45.21 | L5.1 10.22,46.8 12.51,46.8 C6.1 12.76,46.68 12.76,45.59 12.38,45.21 10.41,45.21 | 10.41,45.21 10.42,45.21 C5.1 10.22,43.5 10.22,42.29 11.05,41.47 U$1.1 15.49,41.47 17.65,39.31 17.65,34.35 18.29,33.72 22.92,33.72 23.62,33.02 23.62,32.2 24.19,31.62 26.1,31.62 26.8,32.32
N$5  (via drill 0.6)
  Top 0.254: 6.6,26.67 6.98,26.67 7.56,27.24 U1.2 | R19.1 6.6,25.21 6.6,26.67 | v5.59,26.67 6.6,26.67
  Bottom 0.254: J1.LCD-D2 2.52,27.5 4.13,27.5 4.95,26.67 v5.59,26.67
N$6  (via drill 0.6)
  Top 0.254: U$2.8 19.5,23.68 19.05,24.13 v18.22,24.13 | J2.15 18.01,6.45 16.89,5.33 11.49,5.33 10.61,6.22 10.1,6.73 9.65,7.18 v9.65,23.56
  Bottom 0.254: v18.22,24.13 10.22,24.13 v9.65,23.56
N$7  (via drill 0.6)
  Top 0.254: U$2.9 18.85,21.58 18.99,21.72 18.99,22.99 18.67,23.3 v16.95,23.3 | J2.16 17.53,8.64 17.53,6.6 16.7,5.78 11.81,5.78 11.34,6.26 10.67,6.92 10.29,7.3 10.29,22.61 v10.67,22.99
  Bottom 0.254: v16.95,23.3 10.99,23.3 v10.67,22.99
N$8  (via drill 0.6)
  Top 0.254: U$1.23 18.36,30.3 v18.03,29.97 | 18.92,16.13 18.41,16.64 15.56,16.64 15.05,16.13 14.86,16.13 14.1,16.89 14.1,26.48 17.59,29.97 v18.03,29.97 | v18.03,29.97 17.59,29.97 | U$1.29 21.36,30.33 v21.34,30.3
  Bottom 0.254: L1.1 C10.1 19.43,29.54 19.13,29.23 | 19.13,29.23 19.56,29.23 20.68,28.12 C12.1 | 21.43,28.6 C12.1 | 19.13,29.23 17.31,29.23 C9.1 17.59,29.97 v18.03,29.97 | v21.34,30.3 21.34,28.26 C12.1
N$9  (via drill 0.6)
  Top 0.254: v8.32,23.94 8.32,23.43 9.02,22.73 9.02,6.99 11.18,4.83 17.08,4.83 18.51,6.26 J2.14 | 20.15,24.62 v20.13,24.64 19.94,24.45 19.94,21.72 20.15,21.51 U$2.7
  Bottom 0.254: v8.32,23.94 9.08,24.7 17.53,24.7 17.78,24.95 19.81,24.95 v20.13,24.64
N$10  (via drill 0.6)
  Top 0.254: U$1.49 22.86,46.23 C13.1 C14.1 L2.1 C14.1 v20.38,45.28 | v10.35,40.13 10.69,40.47 U$1.3 12.15,40.47 | U$1.18 15.86,31.17 15.18,30.48 14.09,30.48 C16.1 13.46,30.67 13.46,29.27 13.08,28.89 v11.11,28.89
  Bottom 0.254: v20.38,45.28 20.38,43.24 20.07,42.93 9.78,42.93 9.27,42.42 9.27,40.26 C17.1 v10.35,40.13 10.99,39.5 10.99,38.61 11.11,38.48 v11.11,28.89
N$13
  Top 0.254: 21.59,27.43 23.37,25.65 23.37,22.86 24.13,22.1 24.13,21.34 24.64,20.83
TWI1_SCK  (via drill 0.6)
  Top 0.254: U$1.15 11.94,34.47 | 11.94,34.47 11.48,34.47 10.61,33.59 10.61,32.83 10.29,32.51 7.81,32.51 6.41,33.91 | 6.41,33.91 5.27,35.05 2.58,35.05 J1.TWI1-SCK | v19.37,27.94 19.62,27.69 20.57,27.69 22.86,25.4 22.86,22.35 23.4,21.81 U$2.2 | R3.2 6.23,43.81 v6.1,43.94 | v6.03,33.53 6.41,33.91 | v13.46,32.96 12.51,32.96 11.88,33.59 11.88,34.41 11.94,34.47
  Bottom 0.254: v6.1,43.94 6.1,33.59 v6.03,33.53 | v19.37,27.94 13.91,27.94 13.46,28.39 v13.46,32.96
TWI1_SDA  (via drill 0.6)
  Top 0.254: v18.29,26.92 18.54,27.18 20.32,27.18 22.1,25.4 22.1,22.1 22.75,21.45 U$2.3 | R4.2 5.08,40.45 4.89,40.26 2.59,40.26 J1.TWI1-SDA 2.71,37.47 4.25,37.47 4.83,36.89 4.83,36.51 5.02,36.32 5.97,36.32 7.75,34.54 10.86,34.54 11.28,34.97 U$1.14 14.24,34.97 14.61,34.61 14.86,34.61 15.11,34.35 v15.81,34.35
  Bottom 0.254: v18.29,26.92 13.27,26.92 12.57,27.62 12.57,33.97 12.95,34.35 v15.81,34.35
TX0+
  Top 0.254: J2.7 22.01,10.56 20.15,12.43 U$2.18 20.15,16.56 18.67,18.03 17.14,18.03 16.64,17.53 16,17.53 14.99,18.54 14.99,25.78 17.78,28.58 18.41,28.58 19.36,29.52 U$1.25
TX0-
  Top 0.254: J2.9 21.01,10.87 19.5,12.38 U$2.17 19.5,16.51 18.41,17.59 17.4,17.59 16.89,17.08 15.49,17.08 14.54,18.03 14.54,26.1 17.46,29.02 18.22,29.02 18.86,29.66 U$1.24
TX1+
  Top 0.254: J2.4 23.51,11.03 22.1,12.45 U$2.21 22.1,16.89 21.72,17.27 21.72,17.78 22.1,18.16 24.89,18.16 25.65,18.92 25.65,21.59 25.15,22.1 25.15,22.86 24.38,23.62 24.38,27.18 22.8,28.77 20.89,28.77 20.45,29.21 20.45,30.73 20.86,31.15 U$1.28
TX1-
  Top 0.254: 22.54,8.69 J2.6 22.51,11.34 21.45,12.4 U$2.20 21.45,16.65 20.83,17.27 20.83,18.41 21.08,18.67 24.64,18.67 25.15,19.18 25.15,21.34 24.64,21.84 24.64,22.61 23.88,23.37 23.88,25.91 21.46,28.32 20.45,28.32 20,28.77 20,30.92 20.36,31.29 U$1.27
TX2+
  Top 0.254: J2.1 25.01,11.38 23.4,12.99 U$2.23 23.4,15.52 24,16.13 27.3,16.13 28.19,17.02 28.19,19.69 27.81,20.07 27.43,20.07 27.18,20.32 27.18,22.35 26.67,22.86 26.67,23.62 25.91,24.38 25.91,28.19 23.37,30.73 23.11,30.73 22.36,31.48 U$1.31
TX2-
  Top 0.254: J2.3 24,11.68 22.75,12.94 U$2.22 22.75,15.63 23.69,16.57 26.86,16.57 27.24,16.95 27.24,17.59 26.92,17.91 26.92,18.54 27.05,18.67 27.43,18.67 27.56,18.8 27.56,19.18 27.3,19.43 27.05,19.43 26.67,19.81 26.67,22.1 26.16,22.61 26.16,23.37 25.4,24.13 25.4,27.94 23.11,30.23 22.92,30.23 21.86,31.29 U$1.30
TXC+
  Top 0.254: J2.10 20.51,10.54 18.85,12.21 U$2.16 18.85,15.57 18.22,16.19 15.75,16.19 15.24,15.69 14.61,15.69 13.65,16.64 13.65,26.73 17.86,30.95 U$1.22
TXC-
  Top 0.254: J2.12 19.51,10.78 18.2,12.09 U$2.15 18.2,15.39 17.84,15.75 16.13,15.75 15.49,15.11 14.1,15.11 13.21,16 13.21,26.99 17.34,31.12 17.34,32.19 U$1.21
VCC  (via drill 0.6)
  Top 0.254: L5.2 C7.1 | C7.1 7.37,48.58 | C15.1 L2.2 | 24.38,12.83 24.45,12.76 26.61,12.76 26.54,12.83 | C1.1 26.54,12.83 | 13.16,37.97 U$1.8 15.18,37.97 v15.24,37.91 | U$2.24 24.05,13.16 24.38,12.83 | 24.38,12.83 26.54,12.83 | U$1.35 22.82,34.97 v22.61,35.18 | v15.11,35.43 15.08,35.47 U$1.13 14.51,35.47 | U$1.7 12.27,38.47 v11.81,38.93 11.86,38.97 U$1.6 | U$1.10 15.16,36.97 v15.24,36.89 | U$2.12 16.5,19.95 16.13,20.32 16.13,24.45 v17.08,25.46 | R2.2 8.45,25.27 v8,25.27 7.49,24.77 7.49,23.75 7.05,23.75 R19.2 6.86,23.12 | C15.1 | v8.13,43.62 R3.1 R4.1 8.12,39.69 7.3,38.86 7.11,38.86 6.54,38.29 R1.2 | 26.54,12.83 33.66,12.83 35.56,14.73 37.72,14.73 38.16,15.18 38.16,15.3 38.16,44.83 37.66,45.34 v35.43,45.34 | C7.1 6.26,48.58 v5.65,47.97 | C15.1 14.49,48.45 v14.36,48.32
  Top 0.406: 38.16,7.81 38.16,15.3
  Top 0.61: 6.86,23.12 8,21.98 8,5.14 9.02,4.13 32.13,4.13 35.18,7.18 37.53,7.18 38.16,7.81
  Top 1.016: v32.51,37.85 31.37,38.99 v31.37,42.8
  Bottom 0.254: L1.2 24.38,30.92 C11.1 25.65,30.8 28.38,30.8 28.89,30.29 28.89,29.53 27.81,28.45 26.86,28.45 24.07,25.65 19.24,25.65 19.05,25.46 v17.08,25.46 16.89,25.65 8.38,25.65 v8,25.27 | 22.61,35.88 v22.61,35.18 | J1.VCC3V3 1.25,44.49 2.54,45.85 | 2.54,47.18 3.24,47.82 5.14,47.82 | v5.65,47.97 5.14,47.82 | v14.36,48.32 13.78,47.82 | 13.78,47.82 5.14,47.82 | v8.13,43.62 8.19,43.69 19.11,43.69 19.62,44.2 19.62,45.21 18.54,46.29 | 18.54,46.29 14.35,46.29 14.16,46.48 14.16,47.43 13.78,47.82 | 18.54,46.29 25.27,46.29 26.86,44.7 34.8,44.7 v35.43,45.34
  Bottom 0.61: 2.54,45.85 2.54,47.18
  Bottom 1.016: v15.24,37.91 v15.24,36.89 15.24,35.56 v15.11,35.43 | 22.23,37.91 22.61,37.53 22.61,35.88 | 22.23,37.91 14.08,37.91 13.02,38.97 11.86,38.97 v11.81,38.93 | v31.37,42.8 31.37,44.39 30.99,44.77 | v32.51,37.85 32.45,37.91 22.23,37.91
  pour Bottom (isolate 0.254): 0.13,0 40.89,0 40.89,50 0.13,50
VCC_5V_DCC  (via drill 0.6)
  Top 0.254: v37.34,22.41 28.26,22.41 27.56,23.11 27.56,23.75 26.61,24.7 26.61,26.99 v27.24,27.62 | U$2.11 17.55,21.06 v17.08,21.53
  Bottom 0.254: J1.VCC5V@1 38.1,47.83 38.1,23.05 37.47,22.41 v37.34,22.41 | v27.24,27.62 26.16,26.54 26.16,22.35 25.15,21.34 17.27,21.34 v17.08,21.53 16.45,21.53 16.26,21.34 C3.1
VOUT  (via drill 0.6)
  Top 0.254: POWER_USB.VBUS 31.91,44.54 31.69,44.32 26.86,44.32 26.54,44.64 26.54,46.55 v26.29,46.8
  Bottom 0.254: J1.CHG-IN 24.01,49.08 v26.29,46.8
